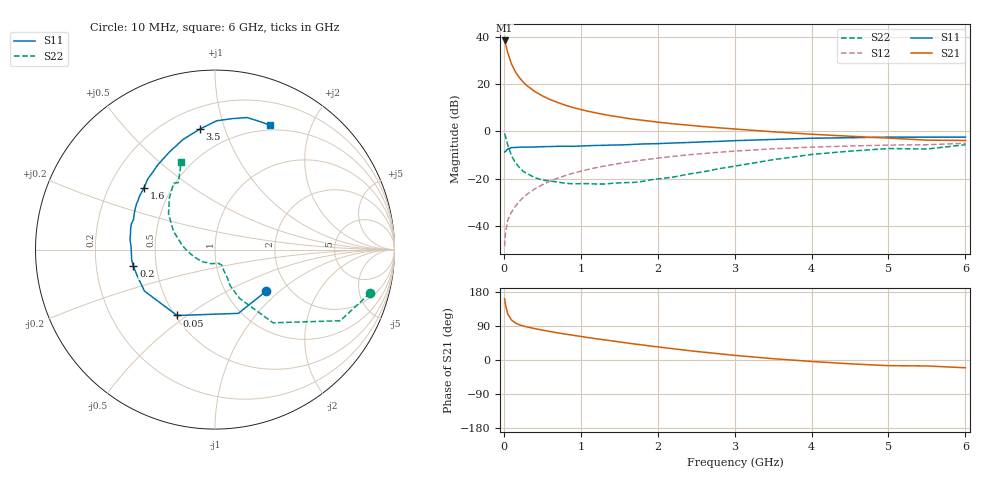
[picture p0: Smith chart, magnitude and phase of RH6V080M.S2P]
! SIEMENS Small Signal Semiconductors
! BFR106
! Si NPN RF Bipolar Junction Transistor in SOT23
! VCE = 6 V  IC = 80 mA
! Common Emitter S-Parameters:  August  1996
# GHz  S  MA  R  50
!  f  S11  S21  S12  S22
! GHz  MAG  ANG  MAG  ANG  MAG  ANG  MAG  ANG
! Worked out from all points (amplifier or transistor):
!   36 points, 10 MHz to 6 GHz, reference 50 ohm
!   highest |S21| = 38.4 dB at 10 MHz (marker M1)
!   |S21| within 3 dB of that: start of sweep to 34.25 MHz
!   unconditionally stable (mu >= 1): 203.6 MHz to 2.333 GHz
!   at 250 MHz: K = 1.03, MAG = 23.3 dB, |S12| = -28.0 dB
!   at 1.4 GHz: K = 1.06, MAG = 8.8 dB, |S12| = -14.1 dB
!   at 6 GHz: K = 0.99, MSG = 0.6 dB, |S12| = -5.0 dB
!   S11 on the Smith chart (normalised r, x): 10 MHz: 1.53, -0.82; 50 MHz: 0.51, -0.46; 200 MHz: 0.37, -0.09; 1.6 GHz: 0.35, +0.33; 3.5 GHz: 0.33, +0.83; 6 GHz: 0.45, +1.44
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0.01  0.3674 -39.0  82.85 161.5  0.0038 82.2  0.8969 -15.7
0.02  0.3783 -69.9  72.91 147.1  0.0069 69.2  0.8025 -29.6
0.05  0.4235 -119.9  46.11 121.5  0.0133 61.8  0.5203 -51.6
0.1  0.4561 -149.6  26.39 105.4  0.0199 63.7  0.3051 -63.2
0.15  0.4579 -162.2  18.09 97.7  0.0264 67.3  0.2191 -67.2
0.2  0.464 -168.5  13.77 93.3  0.0332 70.3  0.1747 -66.3
0.25  0.4679 -173.0  11.06 89.8  0.04 71.0  0.1441 -66.7
0.3  0.4662 -176.8  9.243 87.4  0.0472 72.7  0.1296 -67.2
0.4  0.4683 177.6  7.007 83.0  0.061 73.3  0.1066 -66.8
0.5  0.4768 173.4  5.62 79.0  0.0748 73.2  0.0943 -66.3
0.6  0.4792 169.1  4.708 75.2  0.0893 72.4  0.0897 -68.3
0.8  0.4874 163.0  3.567 68.4  0.1172 70.6  0.0807 -74.3
0.9  0.484 159.6  3.187 65.3  0.1314 69.3  0.0783 -76.7
1.1  0.4993 153.0  2.654 59.0  0.1584 66.9  0.0791 -87.2
1.3  0.5085 147.4  2.276 53.3  0.1852 63.9  0.0777 -96.9
1.6  0.5242 139.1  1.89 44.9  0.224 59.7  0.0834 -114.8
2.2  0.5694 124.1  1.448 29.7  0.2975 51.0  0.1088 -150.3
2.8  0.6171 110.5  1.19 16.4  0.3633 41.8  0.1643 179.0
3.5  0.6767 97.2  0.982 3.5  0.4303 31.4  0.2532 156.1
4.5  0.736 82.5  0.791 -10.1  0.4925 16.8  0.3841 131.4
5.5  0.7562 70.1  0.655 -15.7  0.5232 7.0  0.4256 118.7
6  0.7571 66.0  0.644 -20.5  0.5627 0.0  0.5237 111.1
